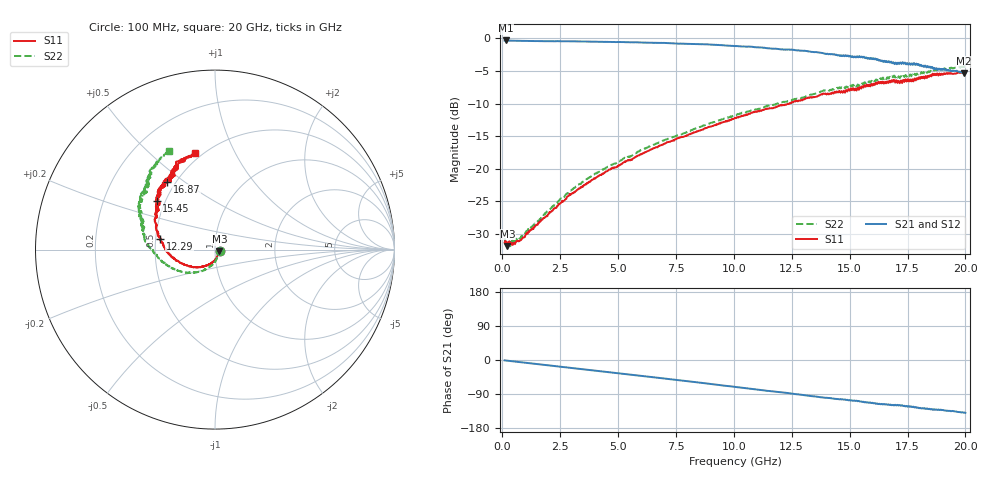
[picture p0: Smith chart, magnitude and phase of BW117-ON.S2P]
!  2-Port S-parameters saved by WinCal
! VAR MeasName=S-Parameters (CALIBRATED_DATA) read from VNA (N5244A)
! VAR MeasDate=11/28/2011 3:34:32 PM
! VAR NAME=240-1
! VAR FILENAME=240-1.S2P
! VAR DATE=11/28/2011 3:34:32 PM
! VAR PHYS_PORTS=1,2
! VAR ObjTypeName=DATASET
! VAR IndexType=Frequency
# Hz S MA R 50
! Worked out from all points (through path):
!   801 points, 100 MHz to 20 GHz, reference 50 ohm
!   highest |S21| = -0.34 dB at 149.8 MHz (marker M1); lowest = -5.3 dB at 19.95 GHz (marker M2)
!   group delay of S21, straight-line fit = 19.6 ps
!   lowest |S11| = -31.8 dB at 224.4 MHz (marker M3), VSWR 1.05, Z = 52.5 - j0.893 ohm
!   |S11| at or under -10 dB: start of sweep to 12.39 GHz
!   |S22| runs from -31.9 to -4.3 dB; largest |S21 - S12| = 0.019
!   S11 on the Smith chart (normalised r, x): 100 MHz: 1.05, -0.01; 12.29 GHz: 0.53, +0.07; 15.45 GHz: 0.45, +0.29; 16.87 GHz: 0.45, +0.43; 20 GHz: 0.46, +0.71
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1e8  0.02716 -11.4  0.96 -1.0  0.96 -1.0  0.0293 -11.1
1.4975e8  0.02785 -10.2  0.9617 -1.4  0.9612 -1.3  0.02661 -14.9
2.24375e8  0.02565 -19.4  0.9595 -1.9  0.96 -1.8  0.02697 -16.8
4.98e8  0.02717 -34.5  0.9554 -3.7  0.9553 -3.7  0.02722 -31.8
8.71125e8  0.02932 -48.5  0.9538 -6.3  0.9537 -6.2  0.03055 -48.7
2.512875e9  0.05456 -87.2  0.9483 -17.5  0.9477 -17.5  0.05906 -84.3
3.43325e9  0.07268 -101.3  0.9448 -23.9  0.9433 -23.8  0.07862 -96.4
4.701875e9  0.1008 -118.0  0.9355 -32.6  0.9356 -32.6  0.1067 -110.2
6.741625e9  0.1486 -138.5  0.9218 -47.0  0.9199 -47.0  0.1585 -127.8
8.856e9  0.2067 -158.9  0.8973 -62.2  0.8961 -62.1  0.2202 -145.6
1.005e10  0.2453 -170.2  0.8721 -71.0  0.875 -70.9  0.2561 -155.7
1.121912e10  0.2803 178.1  0.8489 -79.6  0.8512 -79.3  0.2916 -165.2
1.228875e10  0.3122 168.7  0.8206 -86.9  0.8235 -86.8  0.3268 -174.8
1.338325e10  0.352 157.7  0.7861 -95.4  0.7927 -95.1  0.3704 176.5
1.544788e10  0.4232 140.4  0.7204 -109.7  0.7236 -109.7  0.4464 158.2
1.6219e10  0.4588 133.6  0.6906 -115.9  0.6968 -115.4  0.4839 151.9
1.669162e10  0.4576 128.7  0.6667 -117.5  0.6753 -117.6  0.4927 146.3
1.686575e10  0.4635 125.2  0.6474 -118.3  0.6549 -118.2  0.5027 143.4
1.776125e10  0.4676 120.7  0.6435 -123.1  0.6483 -122.9  0.5115 136.3
1.858212e10  0.5353 114.0  0.5983 -131.2  0.6092 -131.1  0.5695 129.9
1.995025e10  0.5473 101.6  0.5405 -138.8  0.5561 -138.4  0.6094 115.2
2e10  0.55 101.6  0.5434 -139.4  0.558 -138.7  0.6061 114.9
